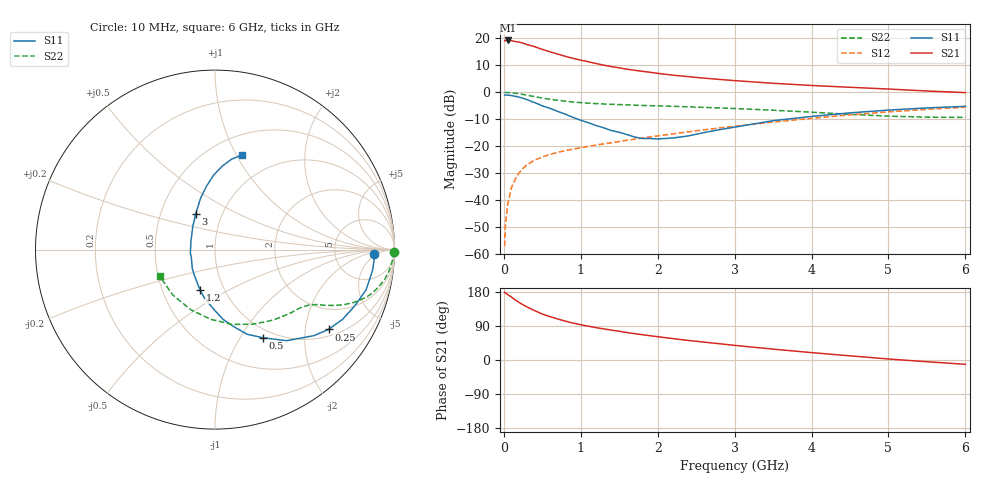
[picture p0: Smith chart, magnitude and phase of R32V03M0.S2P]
! SIEMENS Small Signal Semiconductors
! BFR181
! Si NPN RF Bipolar Junction Transistor in SOT23
! VCE = 2 V  IC = 3 mA
! Common Emitter S-Parameters:  May  1996
# GHz  S  MA  R  50
!  f  S11  S21  S12  S22
! GHz  MAG  ANG  MAG  ANG  MAG  ANG  MAG  ANG
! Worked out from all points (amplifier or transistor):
!   36 points, 10 MHz to 6 GHz, reference 50 ohm
!   highest |S21| = 19.2 dB at 50 MHz (marker M1)
!   |S21| within 3 dB of that: start of sweep to 469.5 MHz
!   unconditionally stable (mu >= 1): 1.326 GHz to 3.177 GHz
!   at 250 MHz: K = 0.31, MSG = 23.2 dB, |S12| = -28.2 dB
!   at 1.4 GHz: K = 1.02, MAG = 13.2 dB, |S12| = -18.7 dB
!   at 6 GHz: K = 0.86, MSG = 2.7 dB, |S12| = -5.5 dB
!   lowest NFmin = 1.40 dB at 450 MHz
!   S11 on the Smith chart (normalised r, x): 10 MHz: 16, -4; 250 MHz: 1.21, -2.67; 500 MHz: 0.88, -1.26; 1.2 GHz: 0.77, -0.37; 3 GHz: 0.75, +0.31; 6 GHz: 0.70, +1.06
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0.01  0.8888 -1.7  9.132 178.7  0.0014 100.5  0.9956 -0.7
0.02  0.8899 -2.8  9.008 177.0  0.0033 85.5  0.9904 -1.4
0.05  0.8854 -7.6  9.137 172.8  0.0084 86.1  0.9904 -3.5
0.1  0.8713 -14.9  9.028 165.9  0.0172 82.3  0.9781 -6.8
0.15  0.8398 -21.9  8.716 158.2  0.0248 77.5  0.9597 -10.0
0.2  0.8098 -28.7  8.509 151.8  0.0322 74.5  0.9352 -12.8
0.25  0.7732 -35.1  8.131 145.6  0.0389 70.8  0.9099 -15.4
0.3  0.7308 -41.0  7.689 140.1  0.0451 68.7  0.8838 -17.5
0.4  0.6451 -51.9  7.004 130.4  0.0552 64.1  0.8302 -20.7
0.5  0.5593 -61.4  6.247 121.2  0.063 61.5  0.7804 -23.2
0.6  0.5048 -69.2  5.629 114.5  0.0704 59.4  0.7402 -24.8
0.8  0.3922 -83.3  4.634 102.6  0.083 57.4  0.6836 -27.0
0.9  0.342 -89.7  4.257 97.4  0.0884 57.2  0.6605 -27.7
1.1  0.272 -103.1  3.67 89.2  0.0995 57.7  0.6282 -29.2
1.2  0.2412 -109.9  3.411 85.3  0.1048 58.0  0.6158 -30.0
1.6  0.1643 -140.4  2.676 72.4  0.1289 58.7  0.5844 -33.3
2.2  0.142 160.8  2.075 56.4  0.1696 59.1  0.5489 -40.2
3  0.2257 118.5  1.645 38.6  0.2341 56.4  0.4996 -52.7
3.5  0.2974 105.7  1.467 28.7  0.2798 53.2  0.4648 -63.5
4.5  0.4151 91.1  1.237 11.0  0.3814 43.7  0.3891 -93.6
5.5  0.5131 79.5  1.056 -4.6  0.4821 31.1  0.3451 -133.0
6  0.5485 74.0  0.986 -11.4  0.5279 23.9  0.3418 -154.2
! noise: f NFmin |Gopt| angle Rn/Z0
0.45  1.4  0.56  17  0.36
0.9  1.5  0.45  35  0.34
1.8  1.85  0.25  82  0.36
